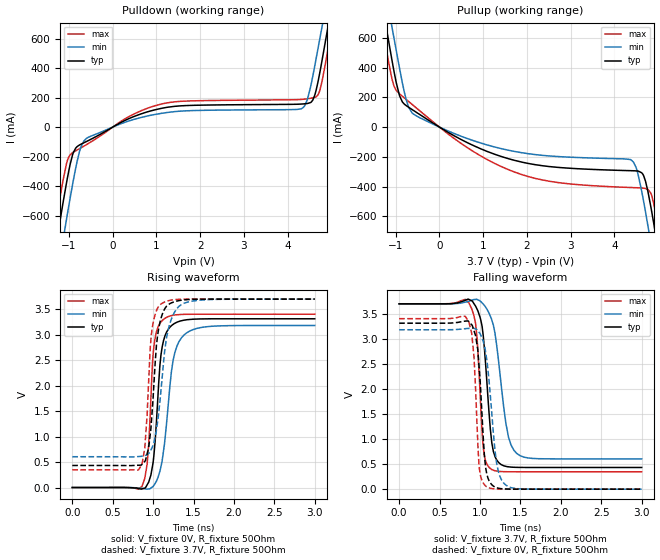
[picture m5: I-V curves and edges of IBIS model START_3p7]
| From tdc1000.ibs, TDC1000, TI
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|   Model
[Model]   START_3p7
Model_type   Output
Polarity   Non-Inverting
Vmeas = 1.85
Vref = 0
Cref = 1pF
Rref = 100000
|   typ   min   max
C_comp   3.839pF   2.875pF   5.918pF
[Voltage Range]   3.7   3.699   3.701
[Temperature Range]   27   125   -40
[Pullup Reference]   3.7   3.699   3.701
[Pulldown Reference]   -0   0   0
[Power Clamp Reference]   3.7   3.699   3.701
[GND Clamp Reference]   0   0   0
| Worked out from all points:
|   slope of the pulldown table from 0 to 0.555 V, typ, clamps not added: 7 ohm
|   slope of the pullup table from 0 to 0.555 V, typ, clamps not added: 6.02 ohm
|   falling waveform, V_fixture 3.7V, R_fixture 50Ohm: 20-80 % time 94.3ps typ, 143ps min, 69.1ps max; typ from 3.7 V to 0.433 V
|   rising waveform, V_fixture 0V, R_fixture 50Ohm: 20-80 % time 90.1ps typ, 132ps min, 69.6ps max; typ from 0 V to 3.31 V
|   rising waveform, V_fixture 3.7V, R_fixture 50Ohm: 20-80 % time 93.7ps typ, 134ps min, 73.2ps max; typ from 0.433 V to 3.7 V
|   falling waveform, V_fixture 0V, R_fixture 50Ohm: 20-80 % time 76.3ps typ, 109ps min, 59.7ps max; typ from 3.31 V to 0 V
[Pulldown]
|   Voltage   I(typ)   I(min)   I(max)
-3.7V     -5.294A    -5.458A    -5.194A
-1.447V   -1.086A    -1.337A    -923.9mA
-1.136V   -515.3mA   -769.8mA   -362.9mA
-902.8mV  -175.7mA   -366.8mA   -170.2mA
-658.6mV  -106mA     -94.3mA    -128.9mA
795.5mV   103.5mA    75.52mA    127.6mA
4.325V    156.6mA    125.9mA    187.9mA
4.581V    184.5mA    348.8mA    198.8mA
4.792V    455.1mA    682.7mA    313mA
4.869V    585.3mA    806.5mA    434.2mA
5.813V    2.172A     2.32A      2.076A
7.4V      4.857A     4.892A     4.849A
[Pullup]
|   Voltage   I(typ)   I(min)   I(max)
-3.7V     4.869A     4.9A       4.865A
-2.102V   2.159A     2.303A     2.068A
-1.191V   625.1mA    838.8mA    481.8mA
-1.091V   457.3mA    679mA      330.8mA
-913.9mV  210.6mA    395.4mA    223.6mA
-625.3mV  117.9mA    94.97mA    152.3mA
1.573V    -211.6mA   -154.8mA   -285.1mA
4.381V    -292.5mA   -219.9mA   -405.7mA
4.658V    -320.1mA   -482.6mA   -409.7mA
4.836V    -538.8mA   -784.2mA   -445.1mA
5.013V    -849.4mA   -1.106A    -696.1mA
7.4V      -5.303A    -5.469A    -5.204A
[Ramp]
R_load = 50
|   typ   min   max
dV/dt_r   1.98819/9.01402e-11   1.90929/1.32458e-10   2.04198/6.95901e-11
dV/dt_f   1.96024/9.42582e-11   1.85671/1.42701e-10   2.01244/6.90816e-11
[Falling Waveform]
V_fixture = 3.7V
V_fixture_min = 3.699V
V_fixture_max = 3.701V
R_fixture = 50Ohm
C_fixture = 0F
|   Time   V(typ)   V(min)   V(max)
0s        3.7V       3.699V     3.701V
863ps     3.788V     3.752V     3.718V
946ps     3.653V     3.788V     3.307V
1.026ns   3.248V     3.718V     1.154V
1.066ns   2.567V     3.642V     579.9mV
1.148ns   915mV      3.37V      390.7mV
1.205ns   589.4mV    2.895V     361.7mV
1.321ns   455.5mV    1.312V     348.6mV
1.454ns   435.5mV    714.1mV    347.1mV
3ns       432.9mV    604.5mV    346.9mV
[Rising Waveform]
V_fixture = 0V
V_fixture_min = 0V
V_fixture_max = 0V
R_fixture = 50Ohm
C_fixture = 0F
|   Time   V(typ)   V(min)   V(max)
0s        4.349uV    26.31uV    2.858uV
863ps     -27.74mV   -16.28mV   23.9mV
925.5ps   50.61mV    -31.33mV   452.3mV
993.9ps   435.1mV    14.8mV     2.48V
1.014ns   709.5mV    51.82mV    2.821V
1.085ns   2.409V     322.5mV    3.224V
1.148ns   2.981V     959.1mV    3.324V
1.248ns   3.204V     2.5V       3.383V
1.42ns    3.295V     3.043V     3.402V
3ns       3.314V     3.182V     3.403V
[Rising Waveform]
V_fixture = 3.7V
V_fixture_min = 3.699V
V_fixture_max = 3.701V
R_fixture = 50Ohm
C_fixture = 0F
|   Time   V(typ)   V(min)   V(max)
0s        432.9mV    604.5mV    346.9mV
863ps     455.7mV    616.5mV    459mV
897.1ps   513.7mV    627.5mV    775.6mV
945.7ps   787.1mV    669.8mV    2.112V
977.1ps   1.251V     749.6mV    2.982V
1.042ns   2.8V       1.134V     3.473V
1.097ns   3.318V     1.901V     3.603V
1.185ns   3.587V     3.086V     3.667V
1.353ns   3.678V     3.596V     3.698V
3ns       3.7V       3.699V     3.701V
[Falling Waveform]
|Gnd
V_fixture = 0V
V_fixture_min = 0V
V_fixture_max = 0V
R_fixture = 50Ohm
C_fixture = 0F
|   Time   V(typ)   V(min)   V(max)
0s        3.314V     3.182V     3.403V
863ps     3.343V     3.209V     3.335V
925.5ps   3.165V     3.21V      2.651V
972.8ps   2.784V     3.163V     941mV
993.9ps   2.342V     3.12V      393.3mV
1.056ns   649.3mV    2.854V     87.9mV
1.082ns   319.3mV    2.604V     47.56mV
1.205ns   28.92mV    530.2mV    3.849mV
1.321ns   3.721mV    80.23mV    395.2uV
3ns       4.341uV    26.28uV    1.942uV
